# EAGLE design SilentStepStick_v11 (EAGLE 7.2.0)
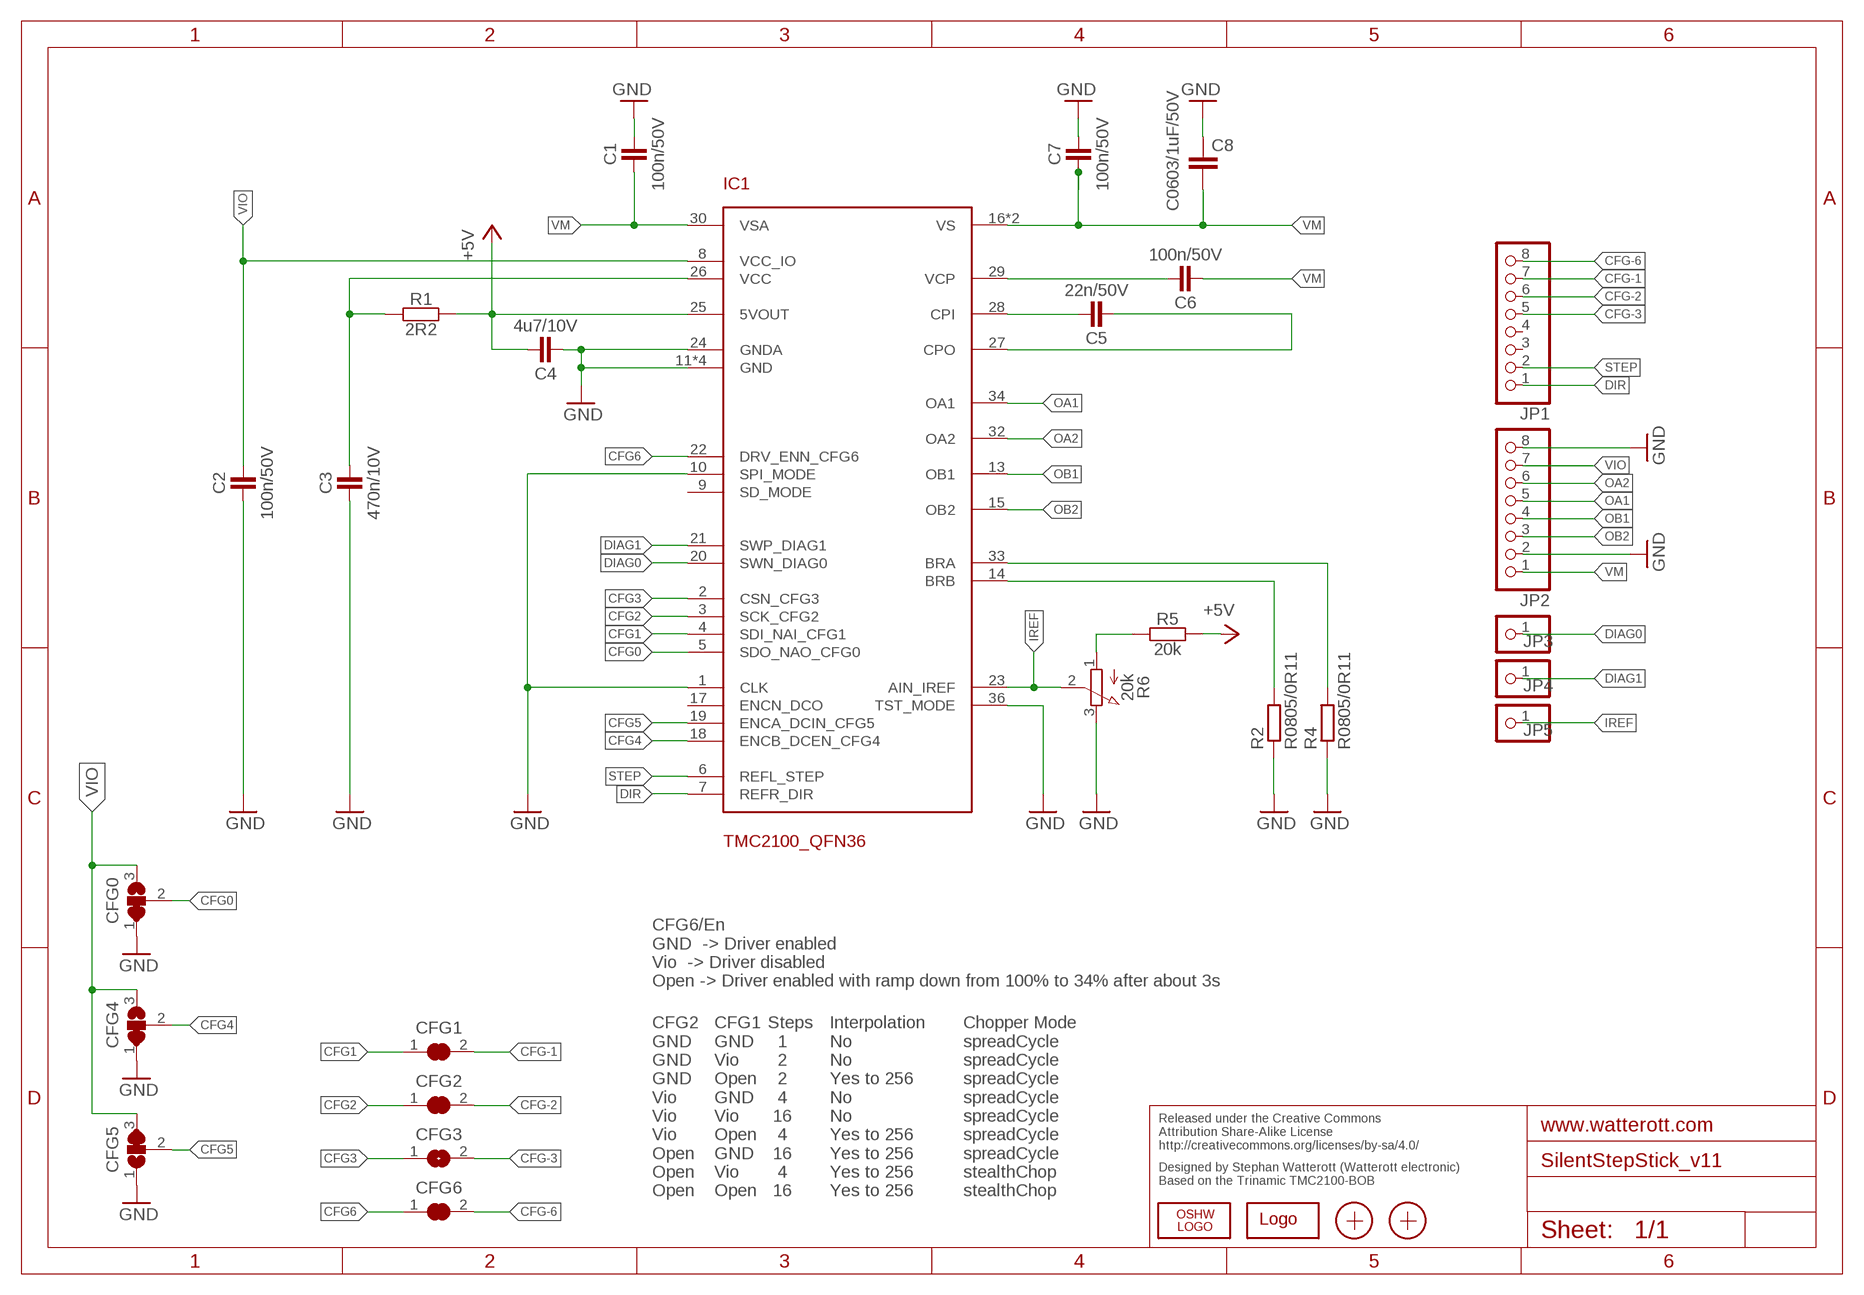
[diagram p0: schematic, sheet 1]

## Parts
C1  100n/50V  CAPACITOR-C0402  [R0402]
C2  100n/50V  CAPACITOR-C0402  [R0402]
C3  470n/10V  CAPACITOR-C0402  [R0402]
C4  4u7/10V  CAPACITOR-C0402  [R0402]
C5  22n/50V  CAPACITOR-C0402  [R0402]
C6  100n/50V  CAPACITOR-C0402  [R0402]
C7  100n/50V  CAPACITOR-C0402  [R0402]
C8  C0603/1uF/50V  C-EUC0603  [C0603]
CFG0  JUMPER3-0201  [JUMPER3-0201]
CFG1  JUMPER2-0201  [JUMPER2-0201]
CFG2  JUMPER2-0201  [JUMPER2-0201]
CFG3  JUMPER2-0201  [JUMPER2-0201]
CFG4  JUMPER3-0201  [JUMPER3-0201]
CFG5  JUMPER3-0201  [JUMPER3-0201]
CFG6  JUMPER2-0201  [JUMPER2-0201]
IC1  TMC2100_QFN36  [QFN36]
JP1  PINHD-1X08_2.54-S  [1X08-S]
JP2  PINHD-1X08_2.54-S  [1X08-S]
JP3  PINHD-1X1  [1X01]
JP4  PINHD-1X1  [1X01]
JP5  PINHD-1X1  [1X01]
LOGO1  OSHW_LOGOX0070  [OSHW_6X70]
LOGO2  LOGO-S_PLACE_M  [SPARK_TPLACE_M]
R1  2R2  RESISTOR-R0402  [R0402]
R2  R0805/0R11  R-EU_M0805  [M0805]
R4  R0805/0R11  R-EU_M0805  [M0805]
R5  20k  RESISTOR-R0402  [R0402]
R6  20k  POTEVM3R  [POT_EVM3R]
X1  PASSER-07  [PASSER_07MM]
X2  PASSER-07  [PASSER_07MM]

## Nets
+5V: C4.2 IC1.25(5VOUT) R1.2 R5.2
CFG0: CFG0.2 IC1.5(SDO_NAO_CFG0)
CFG1: CFG1.1 IC1.4(SDI_NAI_CFG1)
CFG2: CFG2.1 IC1.3(SCK_CFG2)
CFG3: CFG3.1 IC1.2(CSN_CFG3)
CFG4: CFG4.2 IC1.18(ENCB_DCEN_CFG4)
CFG5: CFG5.2 IC1.19(ENCA_DCIN_CFG5)
CFG6: CFG6.1 IC1.22(DRV_ENN_CFG6)
CFG-1: CFG1.2 JP1.7
CFG-2: CFG2.2 JP1.6
CFG-3: CFG3.2 JP1.5
CFG-6: CFG6.2 JP1.8
CPI: C5.2 IC1.28(CPI)
CPO: C5.1 IC1.27(CPO)
DIAG0: IC1.20(SWN_DIAG0) JP3.1
DIAG1: IC1.21(SWP_DIAG1) JP4.1
DIR: IC1.7(REFR_DIR) JP1.1
GND: C1.2 C2.1 C3.1 C4.1 C7.2 C8.2 CFG0.1 CFG4.1 CFG5.1 IC1.1(CLK) IC1.10(SPI_MODE) IC1.11(GND) IC1.12(GND) IC1.24(GNDA) IC1.35(GND) IC1.36(TST_MODE) IC1.GND_PAD(GND) JP2.2 JP2.8 R2.1 R4.1 R6.3(E)
IREF: IC1.23(AIN_IREF) JP5.1 R6.2(S)
N$7: IC1.33(BRA) R4.2
N$9: IC1.14(BRB) R2.2
OA1: IC1.34(OA1) JP2.5
OA2: IC1.32(OA2) JP2.6
OB1: IC1.13(OB1) JP2.4
OB2: IC1.15(OB2) JP2.3
STEP: IC1.6(REFL_STEP) JP1.2
VCC: C3.2 IC1.26(VCC) R1.1
VCP: C6.2 IC1.29(VCP)
VIO: C2.2 CFG0.3 CFG4.3 CFG5.3 IC1.8(VCC_IO) JP2.7
VM: C1.1 C6.1 C7.1 C8.1 IC1.16(VS) IC1.30(VSA) IC1.31(VS) JP2.1
VREF1: R5.1 R6.1(A)
Unconnected: IC1.9(SD_MODE) IC1.17(ENCN_DCO) JP1.3 JP1.4

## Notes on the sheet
- CFG6/En
  GND  -> Driver enabled
  Vio  -> Driver disabled
  Open -> Driver enabled with ramp down from 100% to 34% after about 3s
- CFG2
  GND
  GND
  GND
  Vio
  Vio
  Vio
  Open
  Open
  Open
- CFG1
  GND
  Vio
  Open
  GND
  Vio
  Open
  GND
  Vio
  Open
- Steps
    1
    2
    2
    4
   16
    4
   16
    4
   16
- Interpolation
  No
  No
  Yes to 256
  No
  No
  Yes to 256
  Yes to 256
  Yes to 256
  Yes to 256
- Chopper Mode
  spreadCycle
  spreadCycle
  spreadCycle
  spreadCycle
  spreadCycle
  spreadCycle
  spreadCycle
  stealthChop
  stealthChop
- Released under the Creative Commons
  Attribution Share-Alike License
  http://creativecommons.org/licenses/by-sa/4.0/
- Designed by Stephan Watterott (Watterott electronic) 
  Based on the Trinamic TMC2100-BOB

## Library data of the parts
C1-C7 = we-rcl:CAPACITOR: Capacitors
C8 = rcl:C-EU: CAPACITOR, European symbol
CFG0 CFG4 CFG5 = we-rcl:JUMPER3: 3 Pin Jumpers
CFG1-CFG3 CFG6 = we-rcl:JUMPER2: 2 Pin Jumpers
IC1 = TMC2100_QFN:TMC2100_QFN36
JP1 JP2 = pinhead-2:PINHD-1X08: PIN HEADER
JP3-JP5 = pinhead:PINHD-1X1: PIN HEADER
LOGO1 = we-symbol:OSHW_LOGO: Open-Source-Hardware Logo
LOGO2 = we-symbol:LOGO: Watterott electronic Logo
R1 R5 = we-rcl:RESISTOR: Resistors
R2 R4 = rcl:R-EU_: RESISTOR, European symbol
R6 = we-rcl:POT: Potentiometer
X1 X2 = we-symbol:PASSER: Fiducial Markers

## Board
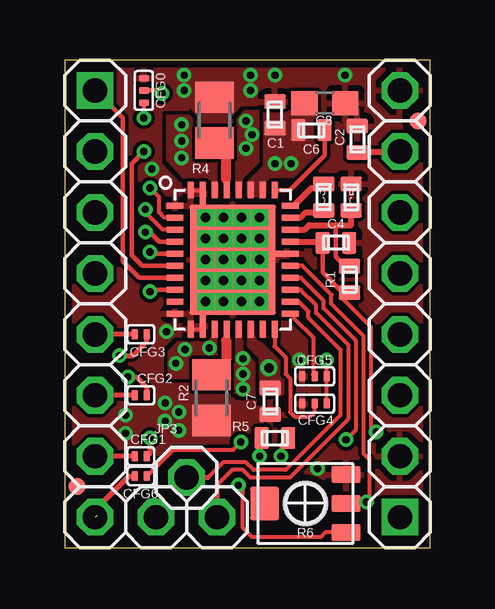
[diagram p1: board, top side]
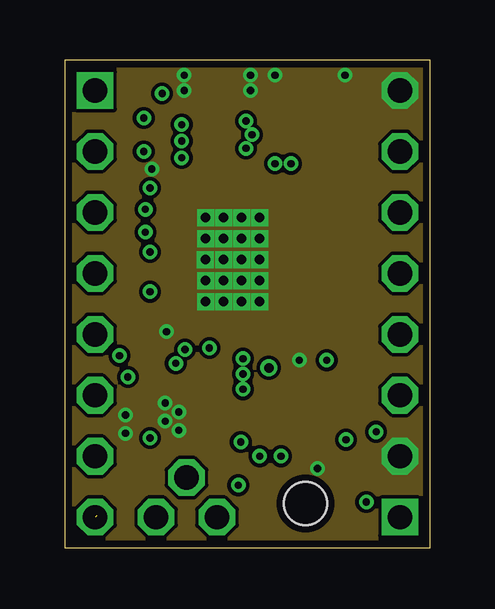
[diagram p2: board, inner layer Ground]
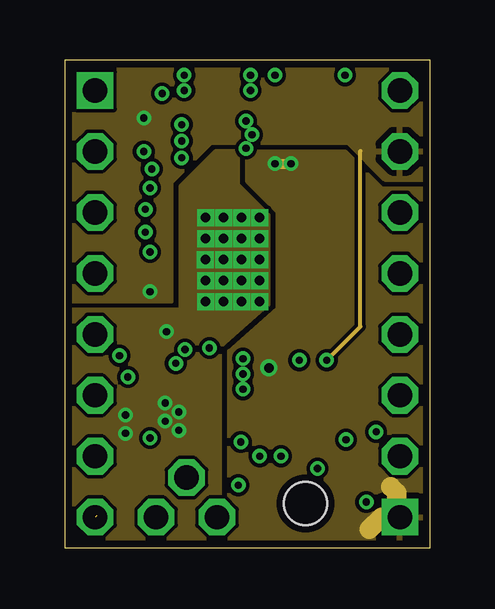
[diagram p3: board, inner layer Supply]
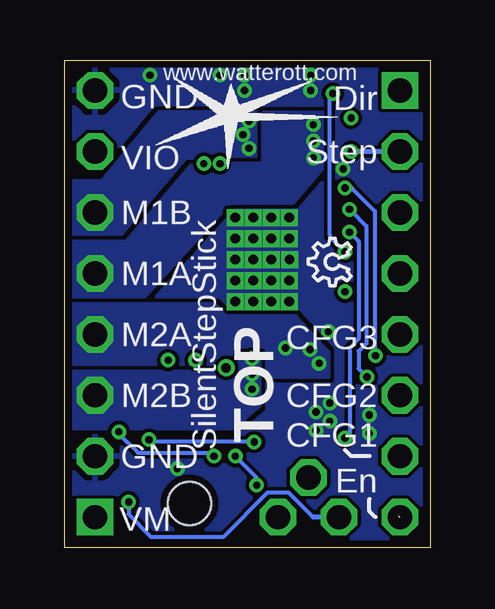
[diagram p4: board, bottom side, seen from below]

Size 15.24 x 20.32 mm. Coordinates in mm from the lower left corner, seen from the top.
Outline: 0,0 15.24,0 15.24,20.32 0,20.32 0,0
Copper layers (1*2*15*16): Top 0.035mm / dielectric 0.36mm / Ground 0.035mm / dielectric 0.71mm / Supply 0.035mm / dielectric 0.2mm / Bottom 0.035mm
Design rules "Default_WE_Euro *": minimum track width 0.15mm, minimum drill 0.25mm, track to track 0.15mm, track to pad 0.15mm, pad to pad 0.15mm, via to via 0.15mm, smd to smd 0mil, copper to edge 0.3mm, drill to drill 8mil, minimum pad ring 10mil, minimum via ring 6mil, stop-mask expansion 2mil, vias tented up to drill 0.5mm, thermal gap 10mil

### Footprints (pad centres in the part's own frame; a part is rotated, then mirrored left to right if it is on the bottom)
R0402 = smd 0.9 x 0.6: 1 0,0.55; 2 0,-0.55
C0603 = smd 1.1 x 1: 1 -0.85,0; 2 0.85,0
JUMPER3-0201 = smd 0.43 x 0.28: 1 0,0.51; 2 0,0; 3 0,-0.51
JUMPER2-0201 = smd 0.43 x 0.28: 1 0,0.255; 2 0,-0.255
QFN36 = smd 0.7 x 0.25: 1 -2.4,2.25; 2 -2.4,1.75; 3 -2.4,1.25; 4 -2.4,0.75; 5 -2.4,0.25; 6 -2.4,-0.25; 7 -2.4,-0.75; 8 -2.4,-1.25; 9 -2.4,-1.75; 10 -2.4,-2.25; 19 2.4,-2.25; 20 2.4,-1.75; 21 2.4,-1.25; 22 2.4,-0.75; 23 2.4,-0.25; 25 2.4,0.75; 26 2.4,1.25; 27 2.4,1.75; 28 2.4,2.25 | smd 0.25 x 0.7: 11 -1.75,-2.9; 13 -0.75,-2.9; 14 -0.25,-2.9; 15 0.25,-2.9; 16 0.75,-2.9; 17 1.25,-2.9; 18 1.75,-2.9; 29 1.75,2.9; 30 1.25,2.9; 31 0.75,2.9; 32 0.25,2.9; 33 -0.25,2.9; 34 -0.75,2.9; 36 -1.75,2.9 | smd 0.25 x 1: 12 -1.25,-2.75; 35 -1.25,2.75 | smd 1 x 0.25: 24 2.25,0.25 | smd 3.6 x 4.6: GND_PAD 0,0
1X08-S = drill 1.016 square: 1 -8.89,0 | drill 1.016 octagon: 2 -6.35,0; 3 -3.81,0; 4 -1.27,0; 5 1.27,0; 6 3.81,0; 7 6.35,0; 8 8.89,0
1X01 = drill 1.016 octagon: 1 0,0
M0805 = smd 1.3 x 1.6: 1 -0.95,0; 2 0.95,0
POT_EVM3R = smd 0.7 x 1.2: 1 -1.2,-1.7; 2 0,-1.7; 3 1.2,-1.7 | smd 1.4 x 1.2: MOUNT 0,1.7 | hole 1.8: 0,0
PASSER_07MM = smd 0.7 x 0.7: X 0,0

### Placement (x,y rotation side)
C1  8.76,18.03 180 top
C2  12.19,17.02 0 top
C3  11.94,14.61 0 top
C4  11.3,12.7 270 top
C5  10.79,14.61 180 top
C6  10.29,17.4 90 top
C7  8.57,6.1 0 top
C8  10.84,18.53 0 top
CFG0  3.3,19.05 0 top
CFG1  3.17,3.81 270 top
CFG2  3.17,6.35 270 top
CFG3  3.17,8.89 270 top
CFG4  10.41,6 90 top
CFG5  10.41,7.14 90 top
CFG6  3.17,2.98 270 top
IC1  7,12 0 top
JP1  1.27,10.16 270 top
JP2  13.97,10.16 90 top
JP3  5.08,2.92 0 top
JP4  6.35,1.27 0 top
JP5  3.81,1.27 0 top
LOGO1  3.3,10.92 90 bottom
LOGO2  8.26,18.03 0 bottom
R1  11.87,11.18 0 top
R2  6.12,6.25 90 top
R4  6.25,17.81 270 top
R5  8.76,4.57 90 top
R6  10.03,1.84 90 top
X1  0.51,2.54 0 top
X2  14.73,17.78 0 top

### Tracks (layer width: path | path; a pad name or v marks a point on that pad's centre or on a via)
+5V  (via drill 0.3 pad 0.41)
  Top 0.16: 9.02,3.99 v9.02,3.81 9.02,4.28 R5.2 | v12.98,4.83 12.78,5.03 12.78,9.2 11.62,10.35 11.62,10.6 11.85,10.6 R1.2 | 10.79,12.66 C4.2 10.72,12.7 10.67,12.75
  Top 0.18: C4.2 10.75,11.47 11.62,10.6
  Top 0.254: IC1.25 10.67,12.75 10.79,12.75
  Bottom 0.16: v9.02,3.81 9.08,3.87 9.1,3.87 9.17,3.95 12.18,3.95 12.98,4.75 v12.98,4.83
CFG0  (via drill 0.3)
  Top 0.18: v4.06,18.92 3.94,19.05 CFG0.2 | IC1.5 3.62,12.25 v3.56,12.32
  Bottom 0.16: 4.19,13.02 4.19,18.8 v4.06,18.92
  Bottom 0.17: 4.19,13.02 4.19,12.95 v3.56,12.32
CFG1  (via drill 0.3)
  Top 0.18: IC1.4 3.95,12.75 3.56,13.14 v3.37,13.14
  Top 0.2: v3.56,4.57 3.56,3.94 CFG1.1
  Bottom 0.16: v3.56,4.57 3.37,4.76 3.37,8.32 2.98,8.7 2.98,12.76 v3.37,13.14
CFG2  (via drill 0.3)
  Top 0.16: IC1.3 4.08,13.25 3.37,13.97 v3.37,14.1
  Top 0.18: CFG2.1
  Top 0.2: v2.64,7.11 2.98,7.11 3.43,6.67 CFG2.1
  Bottom 0.16: v2.64,7.11 v2.63,7.11 2.99,7.46 2.99,8.19 2.67,8.51 2.67,13.4 v3.37,14.1
CFG3  (via drill 0.3)
  Top 0.17: IC1.2 4.16,13.75 3.94,13.97 3.94,14.61 v3.56,14.99
  Top 0.18: CFG3.1
  Top 0.2: v2.29,8 2.86,8 3.43,8.57 CFG3.1
  Bottom 0.16: v2.29,8 2.29,8.04 2.31,8.06 2.31,14.03 3.27,14.99 v3.56,14.99
CFG4
  Top 0.16: IC1.18 8.75,8.39 9.21,7.94 9.21,7.24 9.4,7.05 9.4,5.65 9.59,5.46 10.22,5.46 10.41,5.65 CFG4.2
CFG5
  Top 0.16: IC1.19 9.55,9.75 9.55,9.56 10.35,8.76 10.35,7.21 CFG5.2
CFG6  (via drill 0.3 pad 0.41)
  Top 0.16: CFG6.1 4.51,4.06 7,4.06 v7.34,4.41 | v11.72,4.5 12.13,4.9 12.13,8.64 10.79,9.97 10.79,10.29 9.83,11.25 IC1.22
  Bottom 0.16: v7.34,4.41 11.63,4.41 v11.72,4.5
CFG-1
  Top 0.2: CFG1.2 JP1.7
CFG-2
  Top 0.2: CFG2.2 JP1.6
CFG-3
  Top 0.2: CFG3.2 JP1.5
CFG-6  (1 unrouted)
  Top 0.2: 1.33,1.33 1.33,1.65 2.67,2.98 CFG6.2
CPI
  Top 0.254: IC1.28 9.55,14.25 10.29,14.99 10.63,14.99 C5.2
CPO
  Top 0.254: IC1.27 9.81,13.75 10.03,13.97 10.71,13.97 C5.1
DIAG0
  Top 0.16: 5.97,2.92 6.6,3.56 7.56,3.56 7.87,3.24 9.21,3.24 11.49,5.52 11.49,8.26 10.16,9.59 10.16,9.84 9.75,10.25 IC1.20
  Top 0.2: 5.97,2.92 JP3.1
DIAG1
  Top 0.16: 6.35,2.6 6.99,3.24 7.43,3.24 7.75,2.92 9.37,2.92 11.81,5.36 11.81,8.45 10.48,9.78 10.48,10.1 9.82,10.75 IC1.21
  Top 0.2: 6.35,2.6 JP4.1
DIR
  Top 0.18: JP1.1 2.41,17.91 2.41,11.94 3.1,11.25 IC1.7
GND  (via drill 0.3, 0.4, 0.4 pad 0.41)
  Top 0.16: IC1.11 5.73,9.1 | IC1.36 5.73,14.9
  Top 0.18: IC1.12 5.75,9.12 5.73,9.1 | 5.73,14.9 5.73,14.77 IC1.35
  Top 0.254: IC1.24 8.38,12.25 v8.13,12
  other vias: 4.98,19.68 4.98,19.05 7.75,19.05 4.76,5.65 4.19,6.03 4.19,5.27 4.25,9 5.88,13.75 6.63,13.75 7.38,13.75 8.13,13.75 5.88,12.88 6.63,12.88 7.38,12.88 8.13,12.88 6.63,12 7.38,12 6.63,11.12 5.88,11.12 7.38,11.12 8.13,11.12 5.88,10.25 6.63,10.25 7.38,10.25 7.75,19.68 8.76,19.68 3.63,15.78 8.13,10.25 4.76,4.89 11.68,19.68 2.54,5.52 2.54,4.76 10.54,3.3 9.78,7.81 5.87,12
  pour Top (rank 6): 0,20.32 15.24,20.32 15.24,0 0,0
  pour Ground (no thermals): 0,20.32 15.24,20.32 15.24,0 0,0
  pour Bottom (rank 6): 0,20.32 15.24,20.32 15.24,0 0,0
  pour Top (no thermals): 5.27,20.07 5.27,18.41 5.71,17.91 6.79,17.91 7.24,18.41 7.24,20.07
  pour Top (no thermals): 5.02,4.25 8.19,4.25 8.2,5.82 7.33,5.82 6.99,6.16 5.02,6.16
  pour Supply: 6.29,16.51 4.83,15.05 4.83,9.91 0,9.91 0,0 6.48,0 6.48,8.38 8.51,10.16 8.51,13.84 7.24,15.11 7.24,16.51
IREF  (via drill 0.3)
  Top 0.16: 11.77,1.88 R6.2 | 11.67,1.91 R6.2 | 11.8,1.91 R6.2 | 9.15,11.75 IC1.23 | IC1.23 9.9,11.75 11.11,10.54 11.11,10.16 12.45,8.83 12.45,3.94 12.7,3.68 12.7,2.03 | IC1.23 9.46,11.75
  Top 0.18: 11.8,1.91 v12.57,1.91 12.7,2.03
  Bottom 0.16: 4.89,1.27 5.91,2.29 6.79,2.29 8.64,0.45 11.62,0.45 12.57,1.4 v12.57,1.91
  Bottom 0.2: JP5.1 4.89,1.27
N$7
  Top 0.254: 6.5,16.61 R4.2 | IC1.33 6.75,15.34 6.73,15.37
  Top 0.406: 6.73,15.37 6.73,16.38 R4.2
N$9
  Top 0.16: 6.73,7.81 R2.2
  Top 0.254: IC1.14 6.75,8.66 6.73,8.64
  Top 0.406: 6.73,8.64 6.73,7.81
OA1  (via drill 0.3)
  other vias: 4.88,17.63 4.88,16.24 4.88,16.94
  pour Top (rank 2, no thermals): 6.31,14.69 6.31,16.12 5.25,16.12 5.25,17.94 4.31,17.94 4.31,16.19 5,15.44 6.19,15.44 6.19,14.69
  pour Bottom (rank 3, no thermals): 12.25,10.12 15.25,10.12 15.25,12.75 12.62,12.75 9.88,16 6.94,16 6.94,18.12 4.25,18.12 4.25,16.12 5.75,14.38 8.37,14.38
OA2  (via drill 0.3)
  other vias: 7.81,17.21 7.56,16.64 7.56,17.78
  pour Top (rank 3, no thermals): 8.12,15.83 8.12,18.12 7.25,18.12 7.25,16.12 7.19,16.13 7.19,14.69 7.3,14.73 7.3,15.05
  pour Bottom (rank 4, no thermals): 15.25,13 12.62,13 9.88,16.12 7.12,16.12 7.12,18.13 11.31,18.13 13.69,15.25 15.25,15.25
OB1  (via drill 0.3)
  other vias: 5.02,8.26 6.03,8.32 4.64,7.68
  pour Top (rank 2, no thermals): 6.29,7.11 6.29,9.33 6.22,9.33 6.22,8.76 5.96,8.5 4.75,8.5 4.38,8.12 4.38,7.14
  pour Bottom (rank 2, no thermals): 15.25,10.12 15.19,7.62 8.4,7.62 8.34,8.12 7,8.12 7,7.14 4.25,7.14 4.25,8.12 5.62,9.62 8.5,9.62 9,10.12
OB2  (via drill 0.3)
  other vias: 7.43,7.87 7.43,7.24 7.43,6.6
  pour Top (rank 3, no thermals): 8,6.44 8,7.94 7.3,8.64 7.3,9.31 7.2,9.31 7.2,8.6 7.05,8.45 7.01,6.44
  pour Bottom (no thermals): 15.25,7.31 15.25,5 8.25,5 7.12,5.94 7.12,8.03 7.97,8.03 arc11 7.99,7.31
STEP  (via drill 0.3)
  Top 0.18: v3.3,16.51 2.79,16 2.79,12.19 3.24,11.75 IC1.6
  Bottom 0.2: v3.3,16.51 JP1.2
VCC
  Top 0.16: R1.1 11.77,11.73 11.75,11.75
  Top 0.17: 11.94,14.04 | 11.94,14.04 C3.2
  Top 0.18: 11.3,13.44 11.3,12.13 11.71,11.73
  Top 0.2: 11.81,11.68 11.75,11.75 | 11.71,11.73 R1.1
  Top 0.254: IC1.26 10,13.25 10.19,13.44 11.3,13.44 11.94,13.44 11.94,14.04
VCP
  Top 0.18: IC1.29 9.38,14.9 10.84,16.36 C6.2
VIO  (via drill 0.3)
  Top 0.16: CFG4.3 CFG5.3 v10.92,7.81
  Top 0.18: IC1.8 3.64,10.75 v3.56,10.67 | CFG0.3 v3.3,17.91
  Top 0.254: JP2.7 13.93,16.47 C2.2
  Supply 0.16: 12.32,16.53 12.32,9.21 v10.92,7.81
  Supply 0.18: v3.56,10.67 3.43,10.54
  pour Supply: 15.24,15.36 15.24,20.32 0,20.32 0,10.29 4.45,10.29 4.45,15.24 6.1,16.89 11.81,16.88 13.34,15.36
VM  (via drill 0.3, 0.4)
  Supply 0.406: v8.76,16 v9.44,16
  Supply 0.813: 13.84,1.4 13.84,2.29 13.59,2.54 | 13.84,1.27 13.21,1.27 12.7,0.76
  other vias: 8.51,7.49
  pour Top (no thermals): 7.69,14.69 7.69,15.19 7.76,15.25 8.38,15.88 8.38,15.87 8.38,18.15 10.45,18.15 10.45,16.21 9.72,15.49 8.51,15.49 8.3,15.28 8.3,14.69
  pour Top (no thermals): 7.69,9.31 7.69,8.43 8.18,7.94 8.18,6.44 9.06,6.44 9.06,7.56 7.81,8.81 7.81,9.31
  pour Supply: 15.24,0 6.86,0 6.86,8.19 8.89,9.97 8.89,13.97 7.62,15.24 7.62,16.51 11.68,16.51 13.21,14.99 15.24,14.99
VREF1  (via drill 0.3)
  Top 0.16: v8.13,3.81 8.13,4.59 | R6.1 10.87,0.64 10.67,0.45 7.81,0.45 7.43,0.83 7.43,2.41 v7.24,2.6
  Top 0.254: R5.1 8.14,4.57 8.13,4.59
  Bottom 0.16: v7.24,2.6 7.24,2.92 v8.13,3.81

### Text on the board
bPlace: www.watterott.com | Dir | GND | Step | VIO | M1B | M1A | CFG3 | M2A | CFG2 | M2B | CFG1 | TOP | SilentStepStick | En | GND | VM
Document: Dir | GND | Step | Vio - 3.3-5V | nc | Motor Coil 1-B | nc | Motor Coil 1-A | CFG3 | Motor Coil 2-A | CFG2 | Motor Coil 2-B | CFG1 | GND | En/CFG6 | Vm | VRef | DIAG0 | DIAG1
